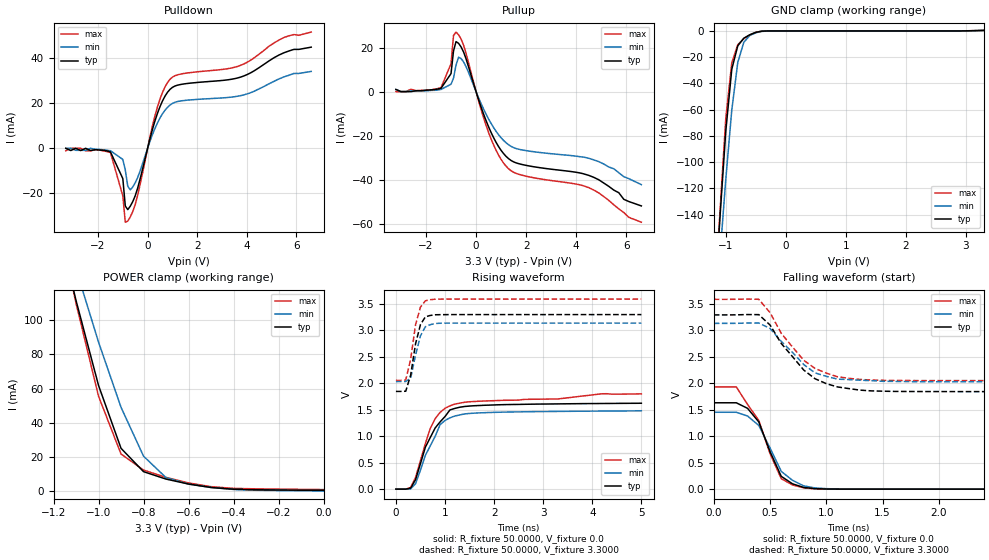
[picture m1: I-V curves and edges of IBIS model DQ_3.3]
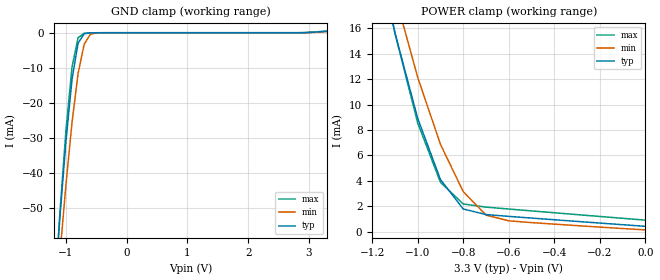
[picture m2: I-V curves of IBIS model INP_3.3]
|*** ISSI Synchronous Sram IBIS Model ***
[IBIS ver]	3.2
[File name]	is61lf204836b165bga.ibs
[File Rev]	1.0
[Date]	May 13,2013
[Notes]
|--- Version History --------------------------------
|1.0: prelimiary
[Disclaimer]	This information is for modeling purpose only
		and is not guaranteed
[Copyright]	INTEGRATED SILICON SOLUTION, INC. 2011
[Component]	IS61LF204836B_165BGA
[Manufacturer]	ISSI
[Package]
| variable   typ   min   max
R_pkg		100.34m			23.84m			218.59m
L_pkg		1.3400nH		0.3700nH		3.0300nH
C_pkg		41.410pF		0.4200pF		150.38pF
[Pin]  signal_name   model_name   R_pin   L_pin   C_pin
R11   A   INP_3.3
R10   A   INP_3.3
R9   A   INP_3.3
R8   A   INP_3.3
R7   TCK   INP_3.3
R6   A0   INP_3.3
R5   TMS   INP_3.3
R4   A   INP_3.3
R3   A   INP_3.3
R2   A   INP_3.3
R1   MODE   INP_3.3
P11   A   INP_3.3
P10   A   INP_3.3
P9   A   INP_3.3
P8   A   INP_3.3
P7   TDO   DQ_3.3
P6   A1   INP_3.3
P5   TDI   INP_3.3
P4   A   INP_3.3
P3   A   INP_3.3
P2   A   INP_3.3
P1   NC   NC
N11   NC   NC
N10   NC   NC
N9   VDDQ   POWER
N8   VSS   GND
N7   NC   NC
N6   A   INP_3.3
N5   NC   NC
N4   VSS   GND
N3   VDDQ   POWER
N2   NC   NC
N1   NC   NC
M11   DQa   DQ_3.3
M10   DQa   DQ_3.3
M9   VDDQ   POWER
M8   VDD   POWER
M7   VSS   GND
M6   VSS   GND
M5   VSS   GND
M4   VDD   POWER
M3   VDDQ   POWER
M2   DQd   DQ_3.3
M1   DQd   DQ_3.3
L11   DQa   DQ_3.3
L10   DQa   DQ_3.3
L9   VDDQ   POWER
L8   VDD   POWER
L7   VSS   GND
L6   VSS   GND
L5   VSS   GND
L4   VDD   POWER
L3   VDDQ   POWER
L2   DQd   DQ_3.3
L1   DQd   DQ_3.3
K11   DQa   DQ_3.3
K10   DQa   DQ_3.3
K9   VDDQ   POWER
K8   VDD   POWER
K7   VSS   GND
K6   VSS   GND
K5   VSS   GND
K4   VDD   POWER
K3   VDDQ   POWER
K2   DQd   DQ_3.3
K1   DQd   DQ_3.3
J11   DQa   DQ_3.3
J10   DQa   DQ_3.3
J9   VDDQ   POWER
J8   VDD   POWER
J7   VSS   GND
J6   VSS   GND
J5   VSS   GND
J4   VDD   POWER
J3   VDDQ   POWER
J2   DQd   DQ_3.3
J1   DQd   DQ_3.3
H11   ZZ   INP_3.3
H10   NC   NC
H9   NC   NC
H8   VDD   POWER
H7   VSS   GND
H6   VSS   GND
H5   VSS   GND
H4   VDD   POWER
H3   NC   NC
H2   VSS   GND
H1   NC   NC
G11   DQb   DQ_3.3
G10   DQb   DQ_3.3
G9   VDDQ   POWER
G8   VDD   POWER
G7   VSS   GND
G6   VSS   GND
G5   VSS   GND
G4   VDD   POWER
G3   VDDQ   POWER
G2   DQc   DQ_3.3
G1   DQc   DQ_3.3
F11   DQb   DQ_3.3
F10   DQb   DQ_3.3
F9   VDDQ   POWER
F8   VDD   POWER
F7   VSS   GND
F6   VSS   GND
F5   VSS   GND
F4   VDD   POWER
F3   VDDQ   POWER
F2   DQc   DQ_3.3
F1   DQc   DQ_3.3
E11   DQb   DQ_3.3
E10   DQb   DQ_3.3
E9   VDDQ   POWER
E8   VDD   POWER
E7   VSS   GND
E6   VSS   GND
E5   VSS   GND
E4   VDD   POWER
E3   VDDQ   POWER
E2   DQc   DQ_3.3
E1   DQc   DQ_3.3
D11   DQb   DQ_3.3
D10   DQb   DQ_3.3
D9   VDDQ   POWER
D8   VDD   POWER
D7   VSS   GND
D6   VSS   GND
D5   VSS   GND
D4   VDD   POWER
D3   VDDQ   POWER
D2   DQc   DQ_3.3
D1   DQc   DQ_3.3
C11   NC   NC
C10   NC   NC
C9   VDDQ   POWER
C8   VSS   GND
C7   VSS   GND
C6   VSS   GND
C5   VSS   GND
C4   VSS   GND
C3   VDDQ   POWER
C2   NC   NC
C1   NC   NC
B11   NC   NC
B10   A   INP_3.3
B9   ADSPB   INP_3.3
B8   OEB   INP_3.3
B7   GWB   INP_3.3
B6   CLK   INP_3.3
B5   BWaB   INP_3.3
B4   BWdB   INP_3.3
B3   CE2   INP_3.3
B2   A   INP_3.3
B1   NC   NC
A11   NC   NC
A10   A   INP_3.3
A9   ADVB   INP_3.3
A8   ADSCB   INP_3.3
A7   BWEB   INP_3.3
A6   CE2B   INP_3.3
A5   BWbB   INP_3.3
A4   BWcB   INP_3.3
A3   CEB   INP_3.3
A2   A   INP_3.3
A1   NC   NC
| Models and submodels in the file (2): DQ_3.3 (3-state), INP_3.3 (Input)
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|   Model DQ_3.3
[Model]		DQ_3.3
Model_type	3-state
Polarity   Non-Inverting
Enable   Active-Low
Vmeas = 	0.7500V
Cref = 		5.0000pF
Rref = 		50.0000
Vref = 		1.2500V
C_comp   3.8290pF   3.3420pF   4.0300pF|
[Temperature Range]	  25.0000   100.0000   0.0
[Voltage Range]   3.3000V   3.1350V   3.6000V
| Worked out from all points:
|   slope of the pulldown table from 0 to 0.495 V, typ, clamps not added: 26.9 ohm
|   slope of the pullup table from 0 to 0.495 V, typ, clamps not added: 31.2 ohm
|   GND clamp passes 1 mA (typ) near -0.49 V on its own axis
|   POWER clamp passes 1 mA (typ) near -0.36 V on its own axis
|   rising waveform, R_fixture 50.0000, V_fixture 0.0: 20-80 % time 480ps typ, 408ps min, 447ps max; typ from 0 V to 1.62 V
|   rising waveform, R_fixture 50.0000, V_fixture 3.3000: 20-80 % time 178ps typ, 175ps min, 176ps max; typ from 1.84 V to 3.29 V
|   falling waveform, R_fixture 50.0000, V_fixture 0.0: 20-80 % time 195ps typ, 217ps min, 242ps max; typ from 1.63 V to 0 V
|   falling waveform, R_fixture 50.0000, V_fixture 3.3000: 20-80 % time 343ps typ, 315ps min, 335ps max; typ from 3.29 V to 1.84 V
[Pulldown]
|Voltage	  I(typ)   I(min)   I(max)
-3.3V     0A         0A         -1.1mA
-1.5V     -1.6mA     -1.08mA    -1.87mA
-1V       -13.48mA   -4.95mA    -21.15mA
-900mV    -25.69mA   -9.639mA   -32.88mA
-800mV    -27.28mA   -16.91mA   -32.39mA
-700mV    -25.77mA   -18.5mA    -30.54mA
-500mV    -21.13mA   -15.36mA   -25.04mA
400mV     15.63mA    11.35mA    18.49mA
900mV     26.18mA    19.21mA    30.66mA
3.7V      31.51mA    23.31mA    36.7mA
5.5V      42.5mA     31.77mA    49.28mA
6.6V      45mA       34.2mA     51.7mA
[Pullup]
|Voltage	  I(typ)   I(min)   I(max)
-3.2V     1mA        900uA      0A
-1.4V     1.5mA      990uA      1.76mA
-1V       8.19mA     3.366mA    12.71mA
-900mV    18.53mA    6.147mA    25.54mA
-800mV    22.75mA    12.11mA    27.08mA
-700mV    21.98mA    15.63mA    25.89mA
-500mV    18.06mA    13.53mA    21.17mA
400mV     -13.22mA   -10.27mA   -15.35mA
1.2V      -29.47mA   -23.28mA   -33.95mA
1.9V      -33.32mA   -26.66mA   -38.21mA
4.5V      -38.1mA    -30.33mA   -43.68mA
6.6V      -52mA      -42.3mA    -59.4mA
[GND_clamp]
|Voltage	  I(typ)   I(min)   I(max)
-3.3V     -1.893A    -1.626A    -2.116A
-1.2V     -220.2mA   -237.3mA   -225.5mA
-1.1V     -144.4mA   -173.5mA   -140.5mA
-1V       -76.37mA   -113.2mA   -66.76mA
-900mV    -29.2mA    -60.35mA   -24.24mA
-800mV    -11.34mA   -23.99mA   -10.52mA
-700mV    -5.573mA   -8.7mA     -5.892mA
-600mV    -2.907mA   -3.457mA   -3.011mA
-500mV    -1.075mA   -1.407mA   -999.8uA
-300mV    -9.492uA   -41.34uA   -5.052uA
3.3V      423.1uA    322.6uA    488.5uA
[POWER_clamp]
|Voltage	  I(typ)   I(min)   I(max)
-3.3V     1.424A     1.197A     1.604A
-1.2V     166.3mA    175.1mA    171.7mA
-1.1V     111.5mA    129.9mA    109.8mA
-1V       61.82mA    87.17mA    55.51mA
-900mV    25.05mA    49.03mA    21.74mA
-800mV    11.41mA    20.46mA    12.33mA
-700mV    7.064mA    7.924mA    8.056mA
-600mV    4.166mA    4.141mA    4.82mA
-500mV    2.143mA    2.162mA    2.625mA
-400mV    1.124mA    995.4uA    1.625mA
0V        423.1uA    141.8uA    910.6uA
[Ramp]
| variable   typ   min   max
dV/dt_r		0.9120/0.3809n   0.7302/0.3836n   1.1604/0.3404n
dV/dt_f		0.8694/0.3076n   0.7542/0.2869n   0.9210/0.3315n
R_load =	50.0000
[Rising Waveform]
R_fixture=	50.0000
V_fixture=	0.0
V_fixture_min=	0.0
V_fixture_max=	0.0
|time   V(typ)   V(min)   V(max)
0s        0V         533.2nV    0V
300ps     18.56mV    3.797mV    30.05mV
400ps     179mV      102.4mV    219.2mV
600ps     791.3mV    638.4mV    860.4mV
700ps     973.8mV    816.1mV    1.144V
900ps     1.268V     1.216V     1.448V
1.1ns     1.494V     1.344V     1.571V
1.4ns     1.559V     1.419V     1.639V
1.9ns     1.585V     1.445V     1.665V
5ns       1.62V      1.476V     1.797V
[Rising Waveform]
R_fixture=	50.0000
V_fixture=	3.3000
V_fixture_min=	3.1350
V_fixture_max=	3.6000
|time   V(typ)   V(min)   V(max)
0s        1.843V     2.029V     2.051V
200ps     1.847V     2.03V      2.057V
300ps     2.15V      2.093V     2.449V
400ps     2.742V     2.529V     3.102V
500ps     3.104V     2.892V     3.434V
600ps     3.25V      3.063V     3.552V
700ps     3.276V     3.103V     3.573V
800ps     3.288V     3.123V     3.583V
1ns       3.291V     3.131V     3.585V
5ns       3.292V     3.131V     3.585V
[Falling Waveform]
R_fixture=	50.0000
V_fixture=	0.0
V_fixture_min=	0.0
V_fixture_max=	0.0
|time   V(typ)   V(min)   V(max)
0s        1.632V     1.453V     1.932V
200ps     1.632V     1.452V     1.931V
300ps     1.527V     1.382V     1.602V
400ps     1.271V     1.204V     1.299V
500ps     710mV      779.4mV    671.9mV
600ps     241.6mV    335.5mV    197.9mV
700ps     100.8mV    166.6mV    80.02mV
800ps     32.06mV    61.86mV    23.86mV
1.2ns     262.2uV    1.546mV    276.4uV
5ns       29.31uV    38.72uV    18.07uV
[Falling Waveform]
R_fixture=	50.0000
V_fixture=	3.3000
V_fixture_min=	3.1350
V_fixture_max=	3.6000
|time   V(typ)   V(min)   V(max)
0s        3.292V     3.132V     3.586V
400ps     3.297V     3.139V     3.587V
500ps     3.102V     3.036V     3.335V
600ps     2.752V     2.791V     2.944V
800ps     2.249V     2.353V     2.434V
900ps     2.087V     2.196V     2.281V
1.1ns     1.931V     2.079V     2.123V
1.3ns     1.871V     2.058V     2.072V
1.6ns     1.847V     2.035V     2.054V
5ns       1.843V     2.029V     2.051V
|   Model INP_3.3
[Model]		INP_3.3
Model_type	Input
Polarity   Non-Inverting
Enable   Active-Low
Vinl = 		0.8000V
Vinh = 		2.0000V
C_comp   3.8290pF   3.3420pF   4.0300pF|
[Temperature Range]	  25.0000   100.0000   0.0
[Voltage Range]   3.3000V   3.1350V   3.6000V
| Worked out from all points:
|   GND clamp passes 1 mA (typ) near -0.73 V on its own axis
|   POWER clamp passes 1 mA (typ) near -0.45 V on its own axis
[GND_clamp]
|Voltage	  I(typ)   I(min)   I(max)
-3.3V     -664.2mA   -601mA     -729.6mA
-1.2V     -76.89mA   -84.89mA   -78.19mA
-1.1V     -52.83mA   -63.46mA   -51.66mA
-1V       -30.98mA   -43.42mA   -27.92mA
-900mV    -13.28mA   -25.61mA   -9.811mA
-800mV    -2.971mA   -11.61mA   -1.401mA
-700mV    -287uA     -3.303mA   -148.3uA
-600mV    -52.18uA   -480.7uA   -48.72uA
-500mV    -11.21uA   -45.78uA   -9.079uA
2.8V      415nA      176.2nA    769.3nA
3.3V      423.1uA    321.5uA    488.5uA
[POWER_clamp]
|Voltage	  I(typ)   I(min)   I(max)
-3.3V     318.3mA    284.6mA    350.6mA
-1.2V     23.85mA    26.22mA    24.49mA
-1.1V     15.64mA    18.66mA    15.62mA
-1V       8.908mA    12.13mA    8.545mA
-900mV    4.097mA    6.862mA    3.88mA
-800mV    1.786mA    3.15mA     2.181mA
-700mV    1.348mA    1.305mA    1.934mA
-600mV    1.205mA    856uA      1.783mA
0V        423.1uA    141.8uA    910.6uA
